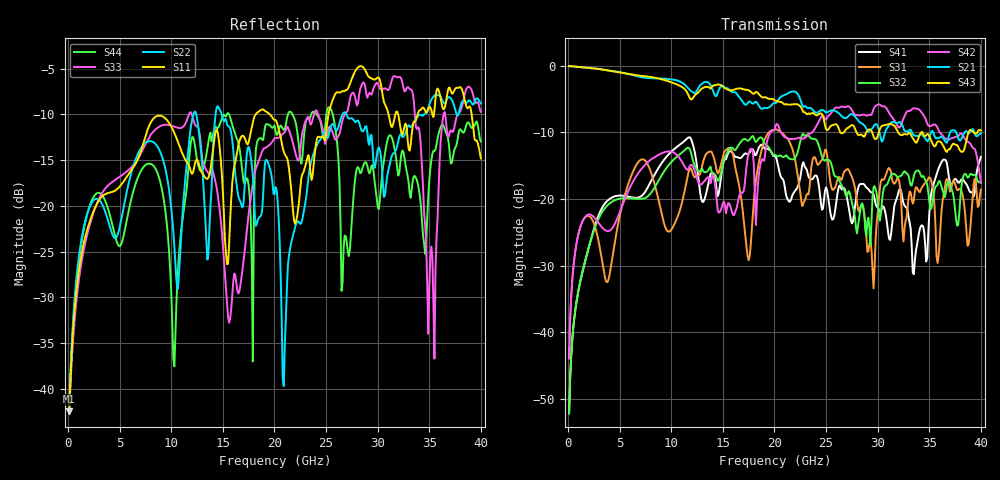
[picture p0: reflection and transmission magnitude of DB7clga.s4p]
! ADC12DJ3200QML-SP
! 196-pin ZMX package
! CLGA Ceramic Package without columns (ceramic land grid array)
! Texas Instruments 4/21/2021
! Single-ended  S-parameters
! PORT#  PORT_NAME  NET_NAME
! PORT1:  DAxN.DIEBUMP DAxN
! PORT2:  DAxN.BGA  DAxN
! PORT3:  DAxP.DIEBUMP DAxP
! PORT4:  DAxP.BGA  DAxP
! Touchstone Ver. 1.0
! Number of ports is 4
# Hz	S	MA	R	50.000000
! SCATTERING PARAMETERS  :
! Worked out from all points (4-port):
!   400 points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, 100 MHz to 40 GHz, reference 50 ohm
!   strongest paths, dB at 100 MHz, 10.1 GHz, 20.1 GHz, 30.1 GHz, 40 GHz:
!     S43: -0.1, -2.5, -5.3, -10.0, -9.7
!     S21: -0.1, -2.1, -5.6, -9.5, -10.1
!     S42: -43.9, -12.9, -9.0, -5.8, -17.5
!     S32: -52.2, -14.3, -13.4, -22.3, -17.6
!     S31: -43.9, -24.4, -9.6, -20.3, -18.6
!     S41: -52.2, -12.8, -13.5, -21.5, -13.7
!   lowest |S11| = -42.5 dB at 100 MHz (marker M1), VSWR 1.02, Z = 50.6 - j0.4 ohm
!   |S11| at or under -10 dB: start of sweep to 18.18 GHz; 19.55 GHz to 25.24 GHz (5.686 GHz wide, 25.4 % of centre); 31.98 GHz to 33.87 GHz (1.888 GHz wide, 5.74 % of centre)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
1e8  0.007539 -31.6  0.9931 -3.4  0.006372 77.0  0.002466 -118.0
     0.9931 -3.4  0.0078 -31.9  0.002467 -118.0  0.006351 77.3
     0.006372 77.0  0.002467 -118.0  0.007337 -28.0  0.993 -3.4
     0.002466 -118.0  0.006351 77.3  0.993 -3.4  0.007618 -28.4
5.3e9  0.1339 -8.3  0.8866 -172.6  0.0936 76.5  0.106 69.1
       0.8866 -172.6  0.09273 -116.5  0.1013 67.9  0.09159 51.2
       0.0936 76.5  0.1013 67.9  0.1481 9.9  0.8849 -171.1
       0.106 69.1  0.09159 51.2  0.8849 -171.1  0.06569 -134.3
1.09e10  0.2046 96.1  0.7576 10.2  0.08576 49.3  0.258 -117.4
         0.7576 10.2  0.05983 -110.0  0.2188 -109.2  0.1975 -63.0
         0.08576 49.3  0.2188 -109.2  0.2664 95.8  0.7031 11.7
         0.258 -117.4  0.1975 -63.0  0.7031 11.7  0.06785 -64.1
1.56e10  0.06087 -126.8  0.6641 -134.7  0.2419 -23.9  0.2268 96.2
         0.6641 -134.7  0.2715 161.9  0.2386 105.5  0.09304 -141.9
         0.2419 -23.9  0.2386 105.5  0.02295 -128.5  0.6546 -125.2
         0.2268 96.2  0.09304 -141.9  0.6546 -125.2  0.3164 -161.9
3.22e10  0.2687 -163.5  0.3758 95.9  0.1164 -71.2  0.1192 -86.3
         0.3758 95.9  0.2458 -138.1  0.149 -62.3  0.3501 -18.1
         0.1164 -71.2  0.149 -62.3  0.5047 -115.9  0.3036 103.9
         0.1192 -86.3  0.3501 -18.1  0.3036 103.9  0.1747 -172.2
3.55e10  0.3309 33.8  0.2979 3.0  0.09076 174.4  0.1354 -130.9
         0.2979 3.0  0.4016 -157.8  0.1163 -158.7  0.3628 -53.5
         0.09076 174.4  0.1163 -158.7  0.01461 59.8  0.2478 10.6
         0.1354 -130.9  0.3628 -53.5  0.2478 10.6  0.1992 -139.5
4e10  0.1817 164.1  0.3116 -119.4  0.1175 -12.8  0.2071 24.3
      0.3116 -119.4  0.3628 155.6  0.1325 57.1  0.1334 -98.8
      0.1175 -12.8  0.1325 57.1  0.3269 -152.7  0.3264 -112.3
      0.2071 24.3  0.1334 -98.8  0.3264 -112.3  0.2246 170.3
